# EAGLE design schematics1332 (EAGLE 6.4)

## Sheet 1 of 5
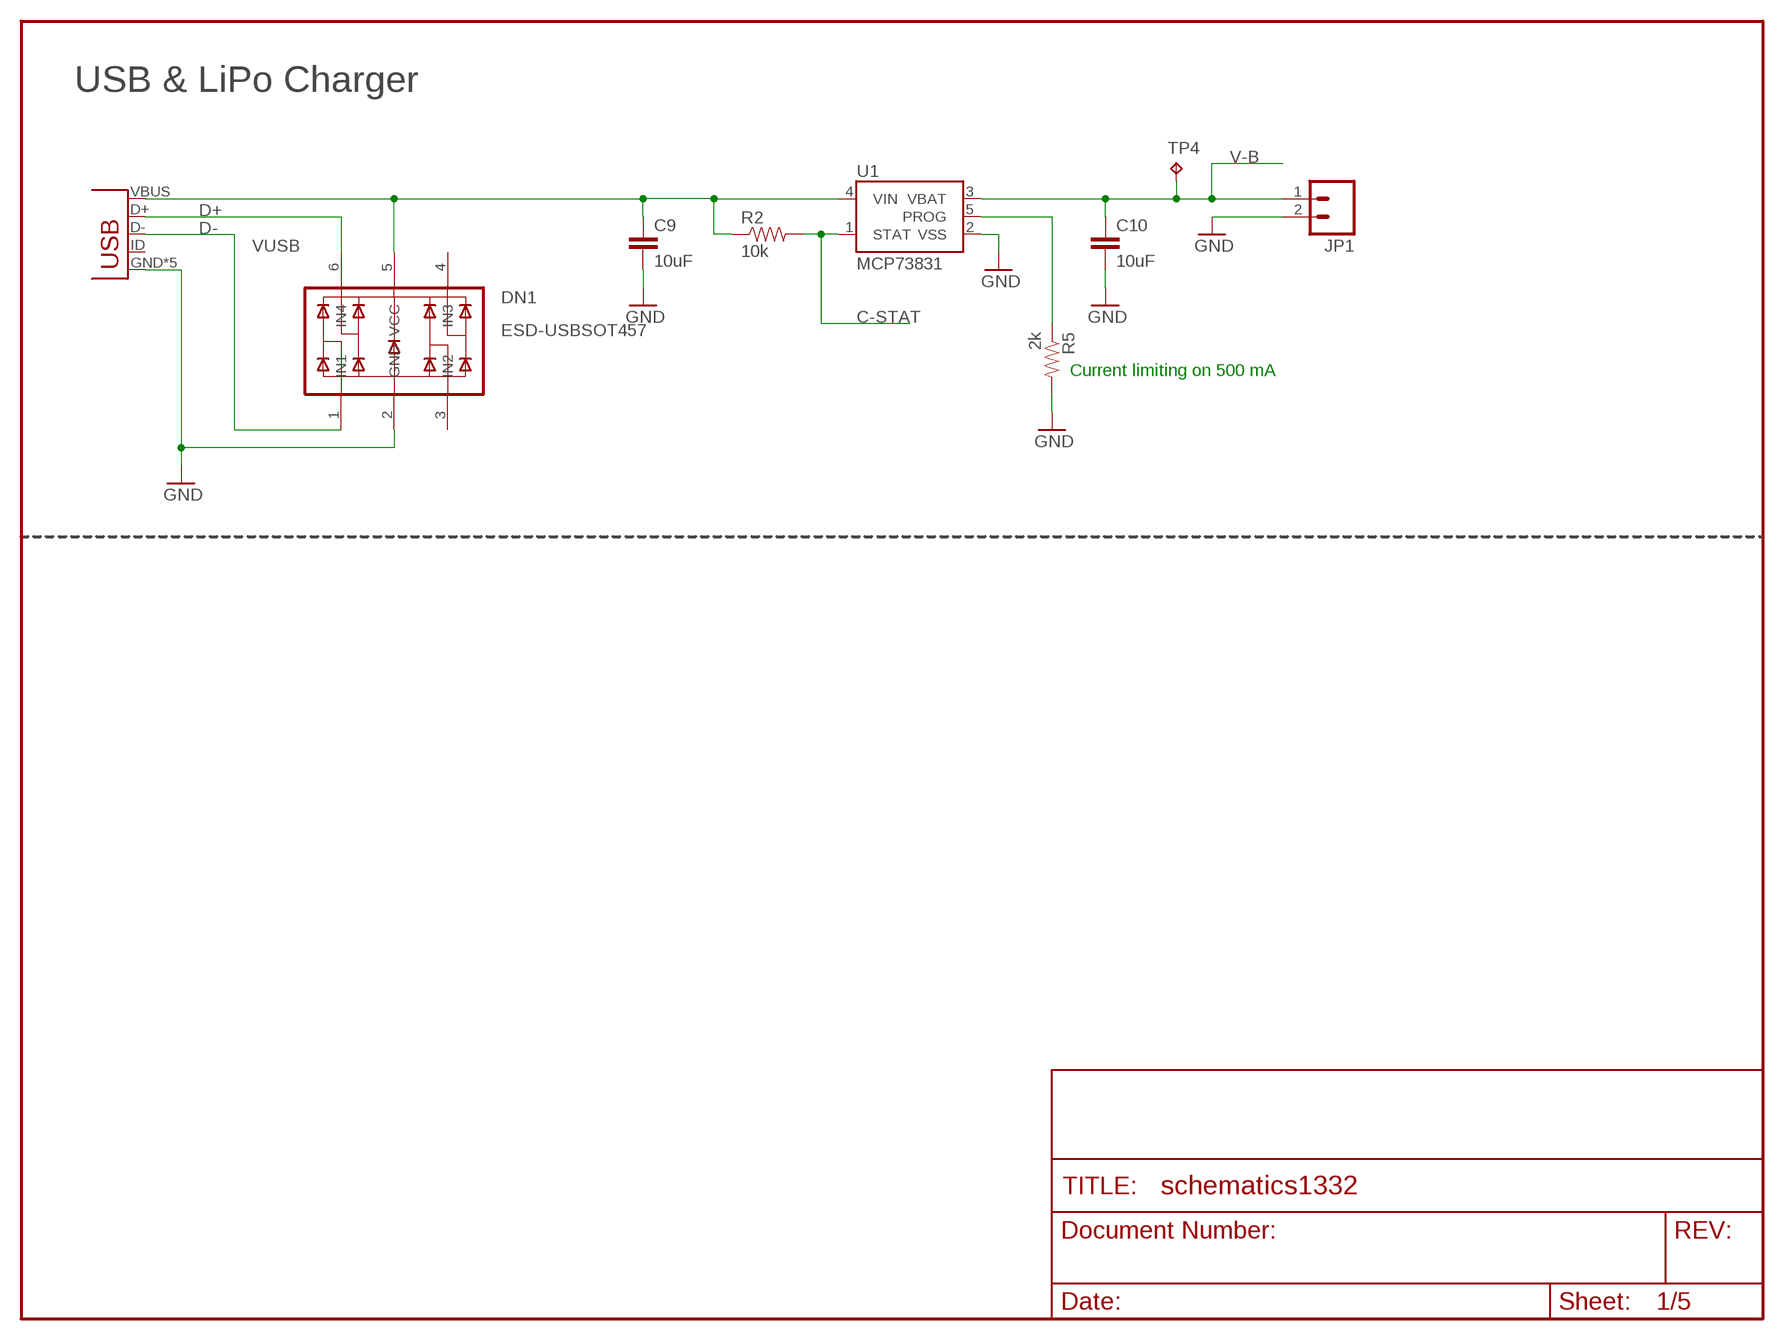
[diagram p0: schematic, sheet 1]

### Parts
C9  10uF  CAP0805  [0805]
C10  10uF  CAP0805  [0805]
DN1  ESD-USBSOT457  [SOT457]
JP1  M02-JST-2MM-SMT  [S2B-PH]
R2  10k  RESISTOR  [0805]
R5  2k  RESISTOR  [0805]
TP4  TPTP20R  [TP20R]
U1  MCP73831  [SOT23-5]
X1  USB  [MICRO-USB-B]

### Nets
C-STAT: R2.2 U1.1(STAT)
D+: DN1.6(IN4) X1.D+ ; also sheet 3
D-: DN1.1(IN1) X1.D- ; also sheet 3
GND: C9.2 C10.2 DN1.2(GND) JP1.2 R5.2 U1.2(VSS) X1.GND X1.GND@1(GND) X1.GND@2(GND) X1.GND@3(GND) X1.GND@4(GND) ; also sheet 2,3,4,5
N$11: R5.1 U1.5(PROG)
V-B: C10.1 JP1.1 TP4.TP U1.3(VBAT) ; also sheet 2
VUSB: C9.1 DN1.5(VCC) R2.1 U1.4(VIN) X1.VBUS ; also sheet 2
Unconnected: DN1.3(IN2) DN1.4(IN3) X1.ID

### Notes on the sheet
- USB & LiPo Charger
- Current limiting on 500 mA

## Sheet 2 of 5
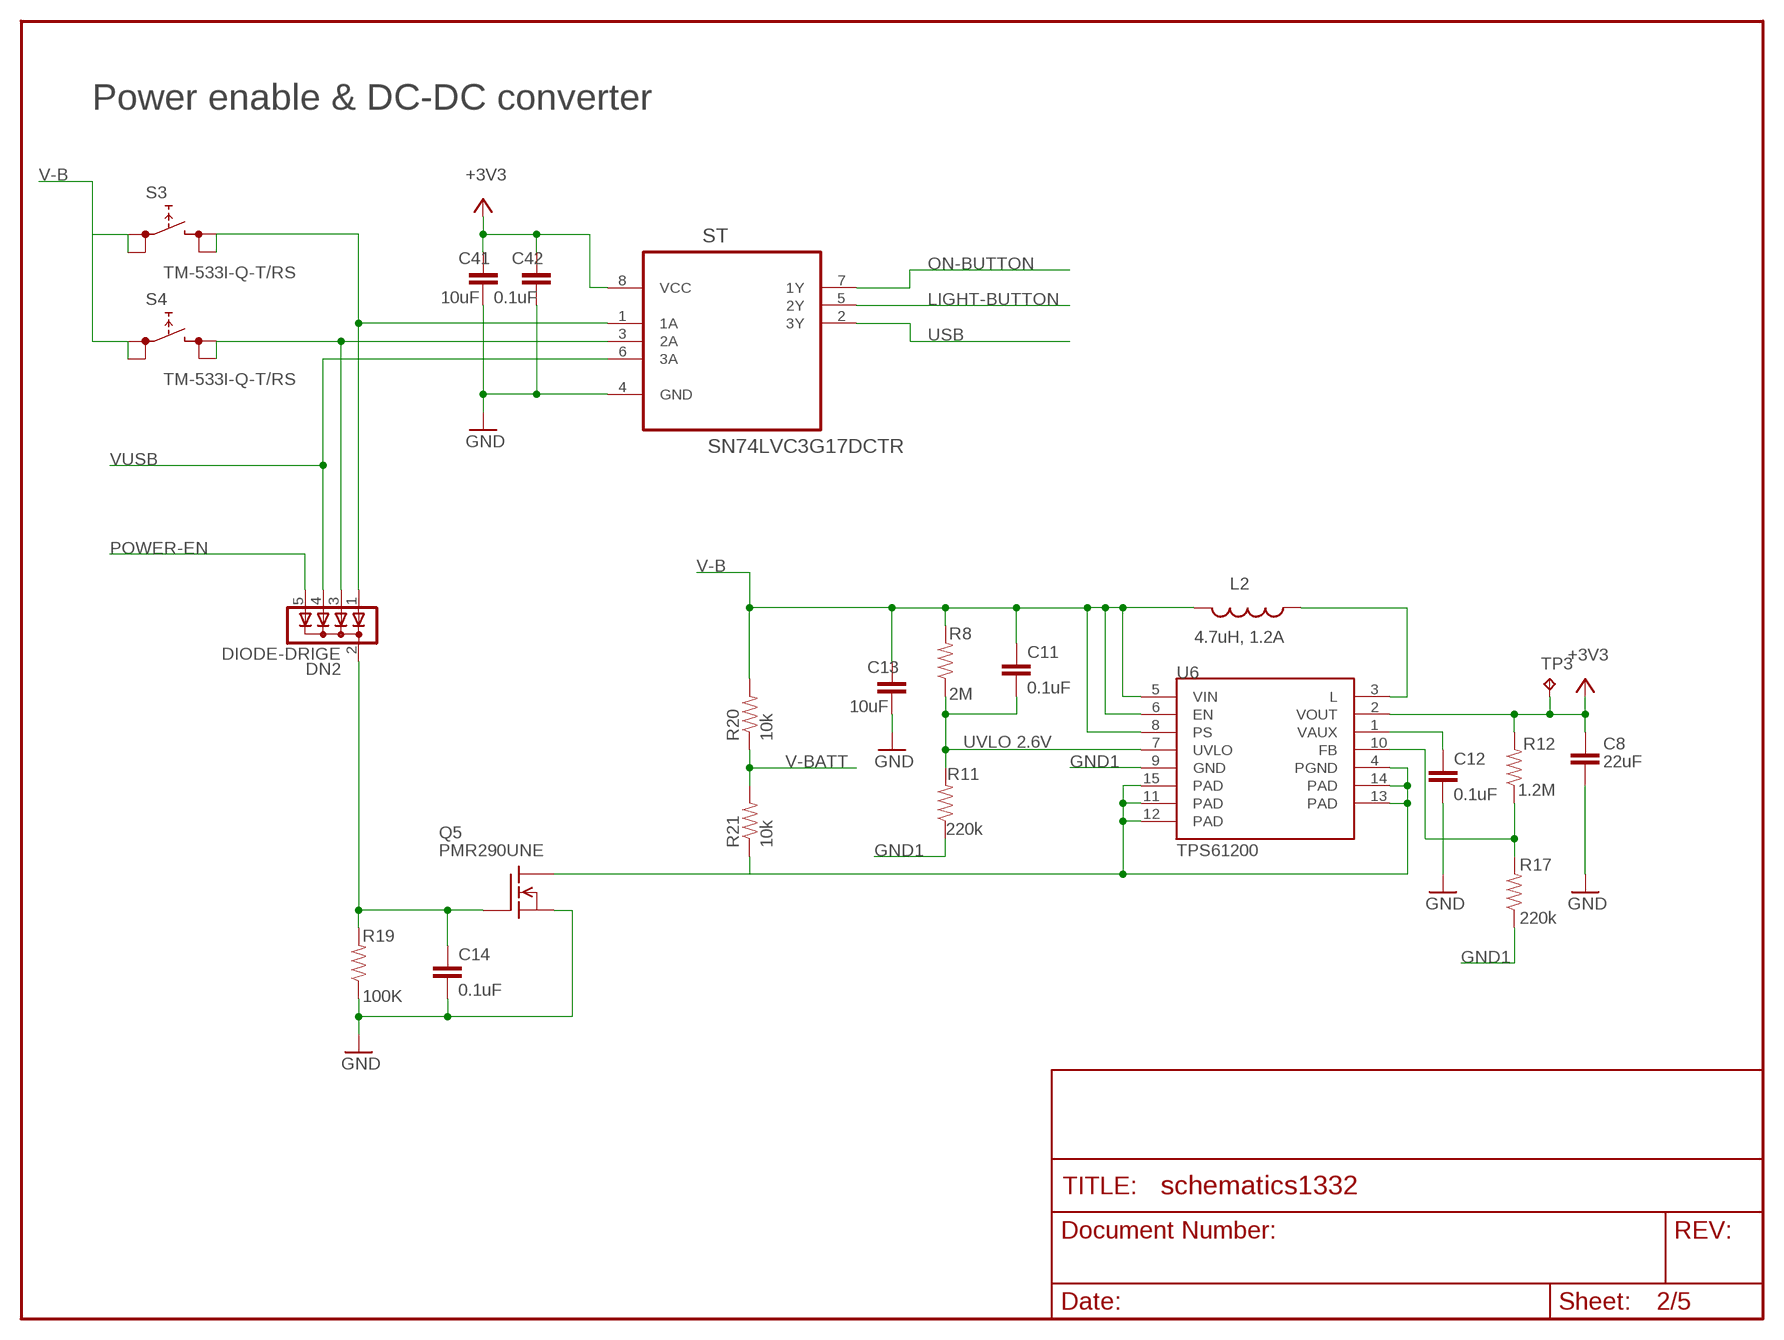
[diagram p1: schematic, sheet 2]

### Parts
C8  22uF  CAP0805  [0805]
C11  0.1uF  CAP0805  [0805]
C12  0.1uF  CAP0805  [0805]
C13  10uF  CAP0805  [0805]
C14  0.1uF  CAP0805  [0805]
C41  10uF  CAP0805  [0805]
C42  0.1uF  CAP0805  [0805]
DN2  DIODE-DRIGE  [SOT353]
L2  4.7uH, 1.2A  INDUCTOR.  [CDRH2D09]
Q5  PMR290UNE  [SOT23]
R8  2M  RESISTOR  [0805]
R11  220k  RESISTOR  [0805]
R12  1.2M  RESISTOR  [0805]
R17  220k  RESISTOR  [0805]
R19  100K  RESISTOR  [0805]
R20  10k  RESISTOR  [0805]
R21  10k  RESISTOR  [0805]
S3  TM-533I-Q-T/RS  [TM-533I-Q-T/R]
S4  TM-533I-Q-T/RS  [TM-533I-Q-T/R]
ST  SN74LVC3G17DCTR  [SOP65P400X130-8N]
TP3  TPTP20R  [TP20R]
U6  TPS61200  [QFN-10_PAD]

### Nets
3.3V1: R12.1 R17.2 U6.10(FB)
+3V3: C8.1 C41.1 C42.1 R12.2 ST.8(VCC) TP3.TP U6.2(VOUT) ; also sheet 3,4,5
GND: C8.2 C12.2 C13.2 C14.2 C41.2 C42.2 Q5.2(S) R19.1 ST.4(GND) ; also sheet 1,3,4,5
GND1: R11.1 R17.1 U6.9(GND)
LIGHT-BUTTON: ST.5(2Y)
LIGHT/WAKEUP-BUTTON1: DN2.3(A2) S4.T3 S4.T4 ST.3(2A)
N$8: L2.P$1 U6.3(L)
N$9: C12.1 U6.1(VAUX)
N$10: C14.1 DN2.2(C) Q5.1(G) R19.2
ON-BUTTON: ST.7(1Y)
PAD@4: Q5.3(D) R21.1 U6.4(PGND) U6.11(PAD) U6.12(PAD) U6.13(PAD) U6.14(PAD) U6.15(PAD)
POWER-EN: DN2.5(A4)
USB: ST.2(3Y)
UVLO1: C11.2 R8.1 R11.2 U6.7(UVLO)
V-B: C11.1 C13.1 L2.P$2 R8.2 R20.2 S3.T1 S3.T2 S4.T1 S4.T2 U6.5(VIN) U6.6(EN) U6.8(PS) ; also sheet 1
V-BATT: R20.1 R21.2 ; also sheet 3
VUSB: DN2.4(A3) ST.6(3A) ; also sheet 1
WAKEUP-BUTTON1: DN2.1(A1) S3.T3 S3.T4 ST.1(1A)

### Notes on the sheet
- Power enable & DC-DC converter
- UVLO 2.6V

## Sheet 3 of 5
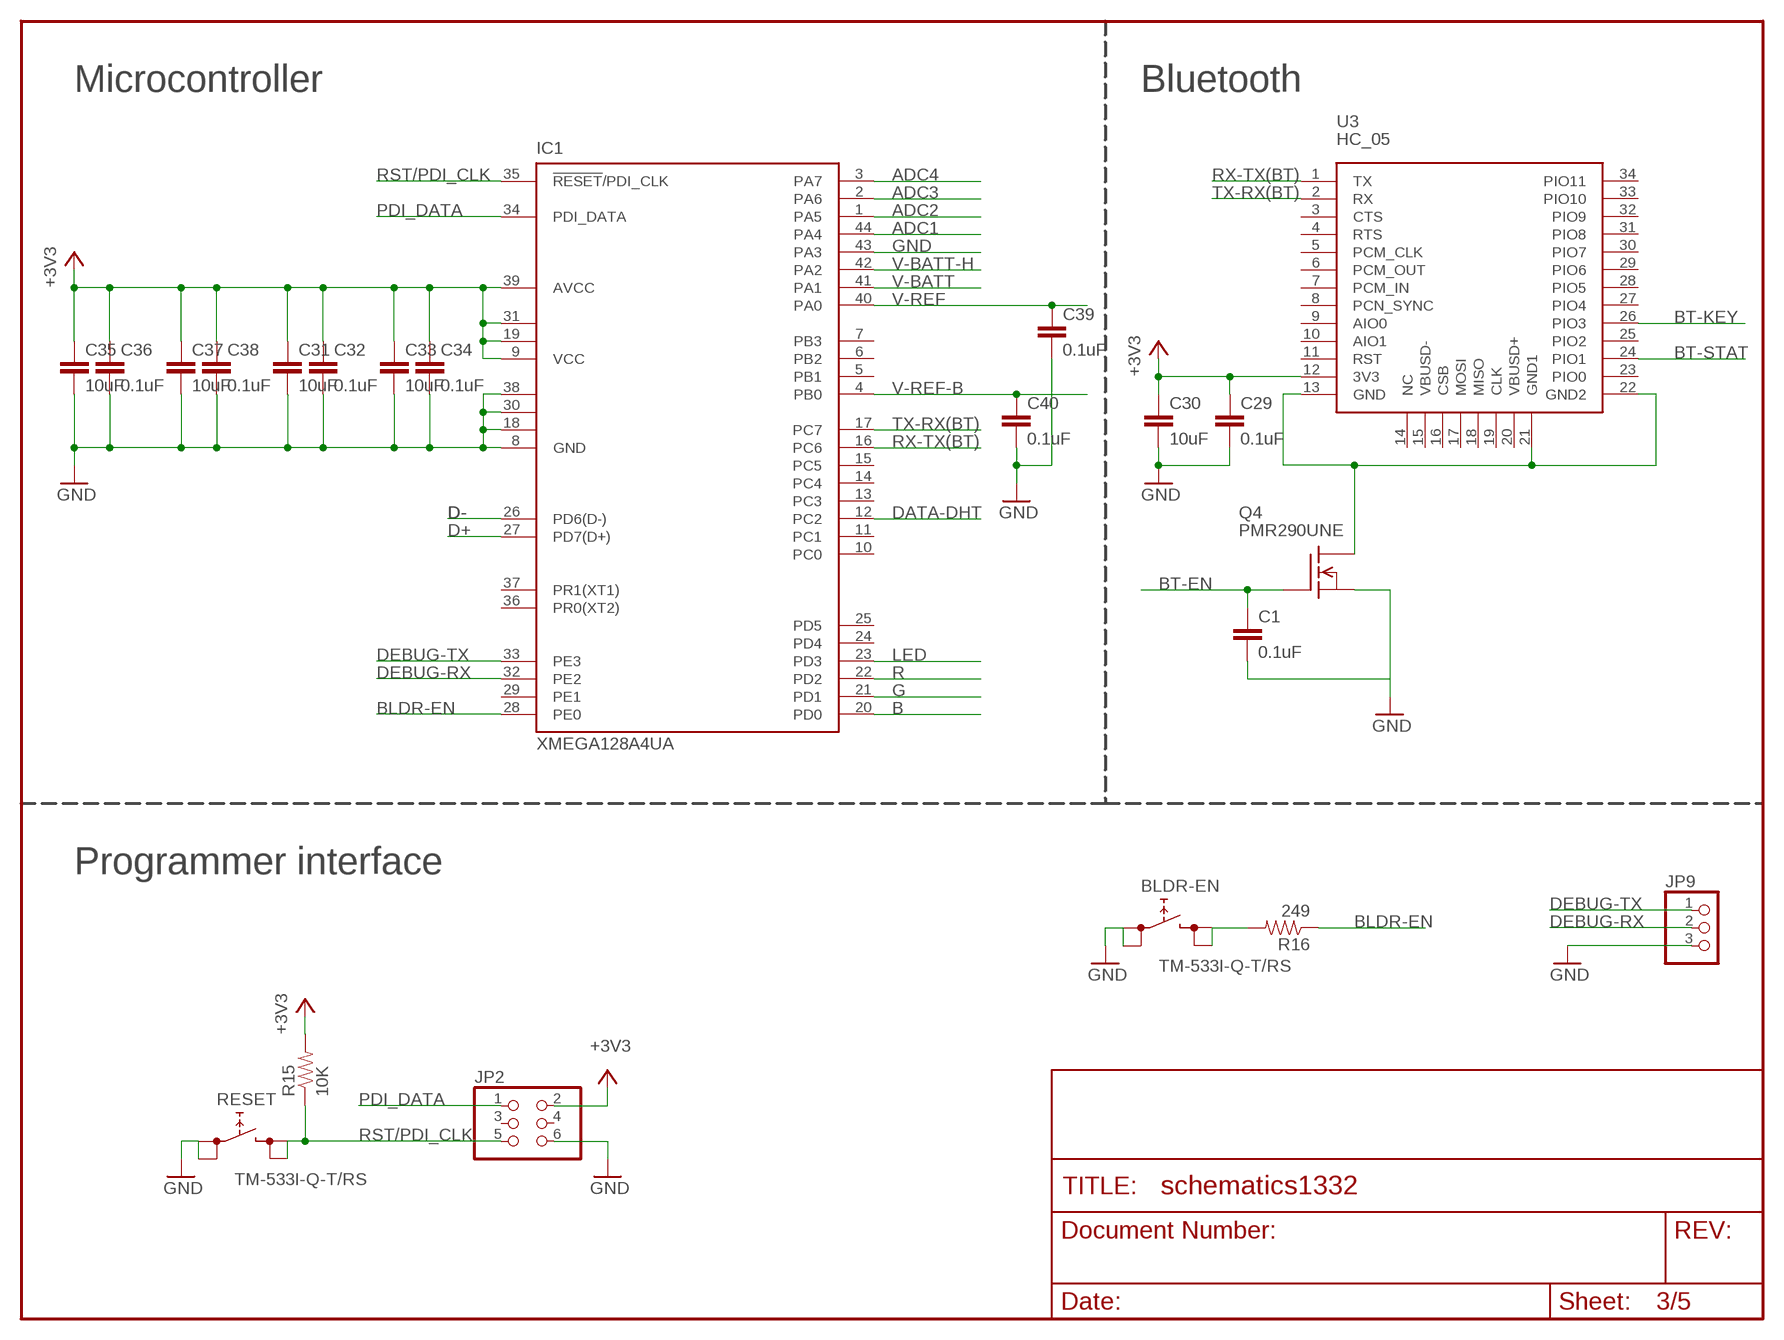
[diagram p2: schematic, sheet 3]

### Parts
BLDR-EN  TM-533I-Q-T/RS  [TM-533I-Q-T/R]
C1  0.1uF  CAP0805  [0805]
C29  0.1uF  CAP0805  [0805]
C30  10uF  CAP0805  [0805]
C31  10uF  CAP0805  [0805]
C32  0.1uF  CAP0805  [0805]
C33  10uF  CAP0805  [0805]
C34  0.1uF  CAP0805  [0805]
C35  10uF  CAP0805  [0805]
C36  0.1uF  CAP0805  [0805]
C37  10uF  CAP0805  [0805]
C38  0.1uF  CAP0805  [0805]
C39  0.1uF  CAP0805  [0805]
C40  0.1uF  CAP0805  [0805]
IC1  XMEGA128A4UA  [TQFP44]
JP2  PINHD-2X3  [2X03]
JP9  PINHD-1X3  [1X03]
Q4  PMR290UNE  [SOT23]
R15  10K  RESISTOR  [0805]
R16  249  RESISTOR  [0805]
RESET  TM-533I-Q-T/RS  [TM-533I-Q-T/R]
U3  HC_05  [BLUETOOTH_SMD]

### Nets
+3V3: C29.1 C30.1 C31.1 C32.1 C33.1 C34.1 C35.1 C36.1 C37.1 C38.1 IC1.9(VCC) IC1.19(VCC1) IC1.31(VCC2) IC1.39(AVCC) JP2.2 R15.2 U3.12(3V3) ; also sheet 2,4,5
ADC1: IC1.44(PA4) ; also sheet 4
ADC2: IC1.1(PA5) ; also sheet 4
ADC3: IC1.2(PA6) ; also sheet 4
ADC4: IC1.3(PA7) ; also sheet 4
B: IC1.20(PD0) ; also sheet 5
BLDR-EN: IC1.28(PE0) R16.1
BT-EN: C1.1 Q4.1(G)
BT-KEY: U3.26(PIO3)
BT-STAT: U3.24(PIO1)
D+: IC1.27(PD7(D+)) ; also sheet 1
D-: IC1.26(PD6(D-)) ; also sheet 1
DATA-DHT: IC1.12(PC2) ; also sheet 5
DEBUG-RX: IC1.32(PE2) JP9.2
DEBUG-TX: IC1.33(PE3) JP9.1
G: IC1.21(PD1) ; also sheet 5
GND: BLDR-EN.T1 BLDR-EN.T2 C1.2 C29.2 C30.2 C31.2 C32.2 C33.2 C34.2 C35.2 C36.2 C37.2 C38.2 C39.2 C40.2 IC1.8(GND) IC1.18(GND1) IC1.30(GND2) IC1.38(GND3) IC1.43(PA3) JP2.6 JP9.3 Q4.2(S) RESET.T1 RESET.T2 ; also sheet 1,2,4,5
LED: IC1.23(PD3) ; also sheet 5
N$4: Q4.3(D) U3.13(GND) U3.21(GND1) U3.22(GND2)
N$5: BLDR-EN.T3 BLDR-EN.T4 R16.2
PDI_DATA: IC1.34(PDI_DATA) JP2.1
R: IC1.22(PD2) ; also sheet 5
RST/PDI_CLK: IC1.35(!RESET!/PDI_CLK) JP2.5 R15.1 RESET.T3 RESET.T4
RX-TX(BT): IC1.16(PC6) U3.1(TX)
TX-RX(BT): IC1.17(PC7) U3.2(RX)
V-BATT: IC1.41(PA1) ; also sheet 2
V-BATT-H: IC1.42(PA2) ; also sheet 4
V-REF: C39.1 IC1.40(PA0) ; also sheet 4
V-REF-B: C40.1 IC1.4(PB0) ; also sheet 4
Unconnected: IC1.5(PB1) IC1.6(PB2) IC1.7(PB3) IC1.10(PC0) IC1.11(PC1) IC1.13(PC3) IC1.14(PC4) IC1.15(PC5) IC1.24(PD4) IC1.25(PD5) IC1.29(PE1) IC1.36(PR0(XT2)) IC1.37(PR1(XT1)) JP2.3 JP2.4 U3.3(CTS) U3.4(RTS) U3.5(PCM_CLK) U3.6(PCM_OUT) U3.7(PCM_IN) U3.8(PCN_SYNC) U3.9(AIO0) U3.10(AIO1) U3.11(RST) U3.14(NC) U3.15(VBUSD-) U3.16(CSB) U3.17(MOSI) U3.18(MISO) U3.19(CLK) U3.20(VBUSD+) U3.23(PIO0) U3.25(PIO2) U3.27(PIO4) U3.28(PIO5) U3.29(PIO6) U3.30(PIO7) U3.31(PIO8) U3.32(PIO9) U3.33(PIO10) U3.34(PIO11)

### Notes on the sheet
- Microcontroller | Bluetooth
- Programmer interface

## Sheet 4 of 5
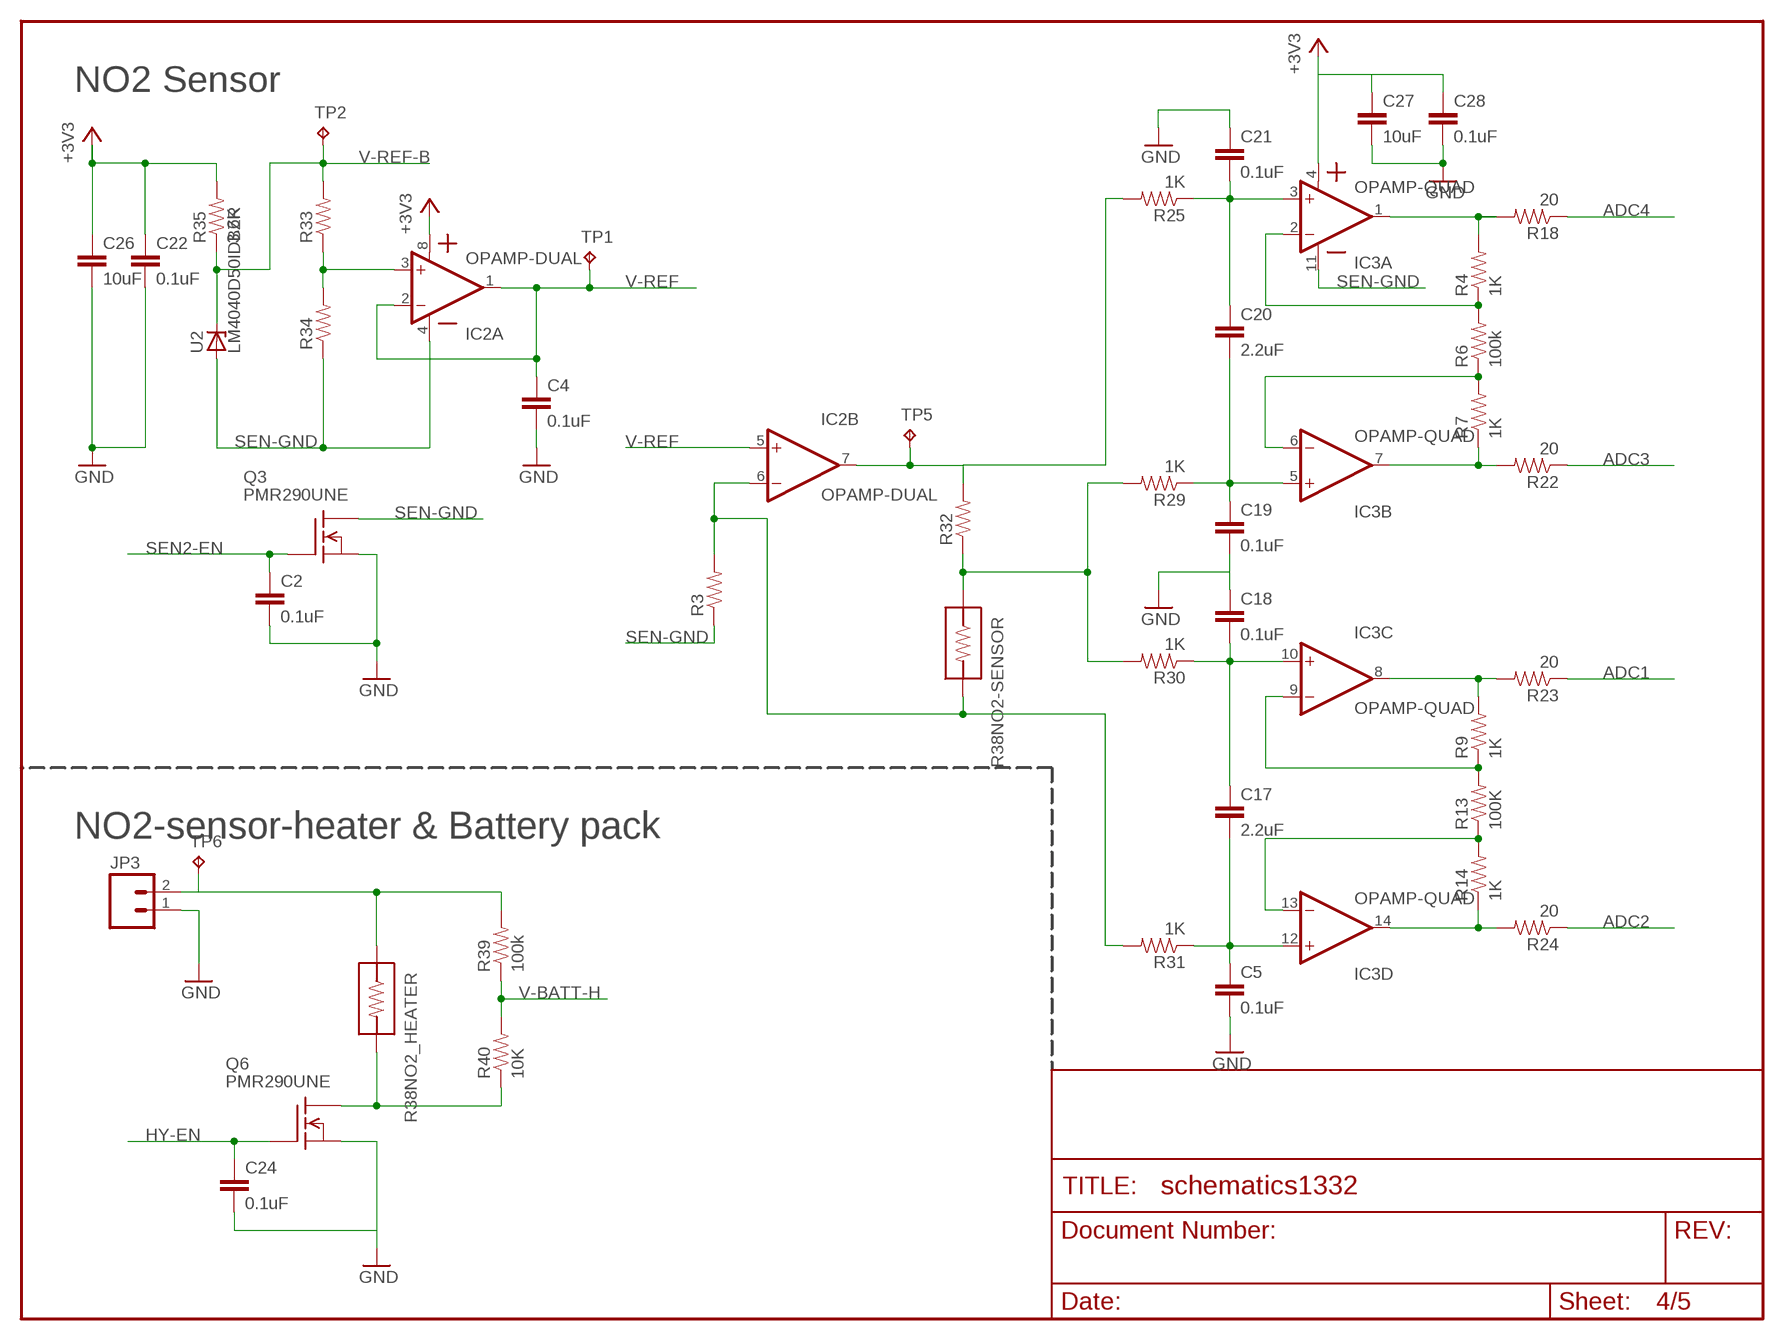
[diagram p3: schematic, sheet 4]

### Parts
C2  0.1uF  CAP0805  [0805]
C4  0.1uF  CAP0805  [0805]
C5  0.1uF  CAP0805  [0805]
C17  2.2uF  CAP0805  [0805]
C18  0.1uF  CAP0805  [0805]
C19  0.1uF  CAP0805  [0805]
C20  2.2uF  CAP0805  [0805]
C21  0.1uF  CAP0805  [0805]
C22  0.1uF  CAP0805  [0805]
C24  0.1uF  CAP0805  [0805]
C26  10uF  CAP0805  [0805]
C27  10uF  CAP0805  [0805]
C28  0.1uF  CAP0805  [0805]
IC2  OPAMP-DUAL  [SOIC127P600X175-8N]
IC3  OPAMP-QUAD  [SOIC127P600X175-14N]
JP3  M025MM  [SCREWTERMINAL-5MM-2]
Q3  PMR290UNE  [SOT23]
Q6  PMR290UNE  [SOT23]
R3  RESISTOR  [0805]
R4  1K  RESISTOR  [0805]
R6  100k  RESISTOR  [0805]
R7  1K  RESISTOR  [0805]
R9  1K  RESISTOR  [0805]
R13  100K  RESISTOR  [0805]
R14  1K  RESISTOR  [0805]
R18  20  RESISTOR  [0805]
R22  20  RESISTOR  [0805]
R23  20  RESISTOR  [0805]
R24  20  RESISTOR  [0805]
R25  1K  RESISTOR  [0805]
R29  1K  RESISTOR  [0805]
R30  1K  RESISTOR  [0805]
R31  1K  RESISTOR  [0805]
R32  RESISTOR  [0805]
R33  RESISTOR  [0805]
R34  RESISTOR  [0805]
R35  3.6K  RESISTOR  [0805]
R38  NO2-SENSOR  [DIP08]
R39  100k  RESISTOR  [0805]
R40  10K  RESISTOR  [0805]
TP1  TPTP20R  [TP20R]
TP2  TPTP20R  [TP20R]
TP5  TPTP20R  [TP20R]
TP6  TPTP20R  [TP20R]
U2  LM4040D50IDBZR  [SOT95P237X112-3N]

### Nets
+3V3: C22.1 C26.1 C27.1 C28.1 IC2.8(A:VDD) IC3.4(A:VDD) R35.2 ; also sheet 2,3,5
ADC1: R23.1 ; also sheet 3
ADC2: R24.1 ; also sheet 3
ADC3: R22.1 ; also sheet 3
ADC4: R18.1 ; also sheet 3
GND: C2.2 C4.2 C5.2 C18.1 C19.2 C21.1 C22.2 C24.2 C26.2 C27.2 C28.2 JP3.1 Q3.2(S) Q6.2(S) ; also sheet 1,2,3,5
HY-EN: C24.1 Q6.1(G)
N$1: IC3.2(A:-IN) R4.1 R6.2
N$2: IC3.6(B:-IN) R6.1 R7.2
N$7: IC3.9(C:-IN) R9.1 R13.2
N$12: IC3.13(D:-IN) R13.1 R14.2
N$14: IC3.1(A:OUT) R4.2 R18.2
N$15: IC3.7(B:OUT) R7.1 R22.2
N$19: IC3.8(C:OUT) R9.2 R23.2
N$21: IC3.14(D:OUT) R14.1 R24.2
N$22: C17.1 C18.2 IC3.10(C:+IN) R30.1
N$23: IC2.3(A:+IN) R33.1 R34.2
N$25: C19.1 C20.2 IC3.5(B:+IN) R29.1
N$26: C20.1 C21.2 IC3.3(A:+IN) R25.1
N$27: C5.1 C17.2 IC3.12(D:+IN) R31.1
N$28: JP3.2 R38.2 R39.2 TP6.TP
N$29: Q6.3(D) R38.7 R40.1
N$33: R29.2 R30.2 R32.1 R38.1
N$34: IC2.7(B:OUT) R25.2 R32.2 TP5.TP
N$35: IC2.6(B:-IN) R3.2 R31.2 R38.8
SEN2-EN: C2.1 Q3.1(G)
SEN-GND: IC2.4(A:GND) IC3.11(A:GND) Q3.3(D) R3.1 R34.1 U2.2(A)
V-BATT-H: R39.1 R40.2 ; also sheet 3
V-REF: C4.1 IC2.1(A:OUT) IC2.2(A:-IN) IC2.5(B:+IN) TP1.TP ; also sheet 3
V-REF-B: R33.2 R35.1 TP2.TP U2.1(C) ; also sheet 3

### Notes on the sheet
- NO2 Sensor
- NO2-sensor-heater & Battery pack

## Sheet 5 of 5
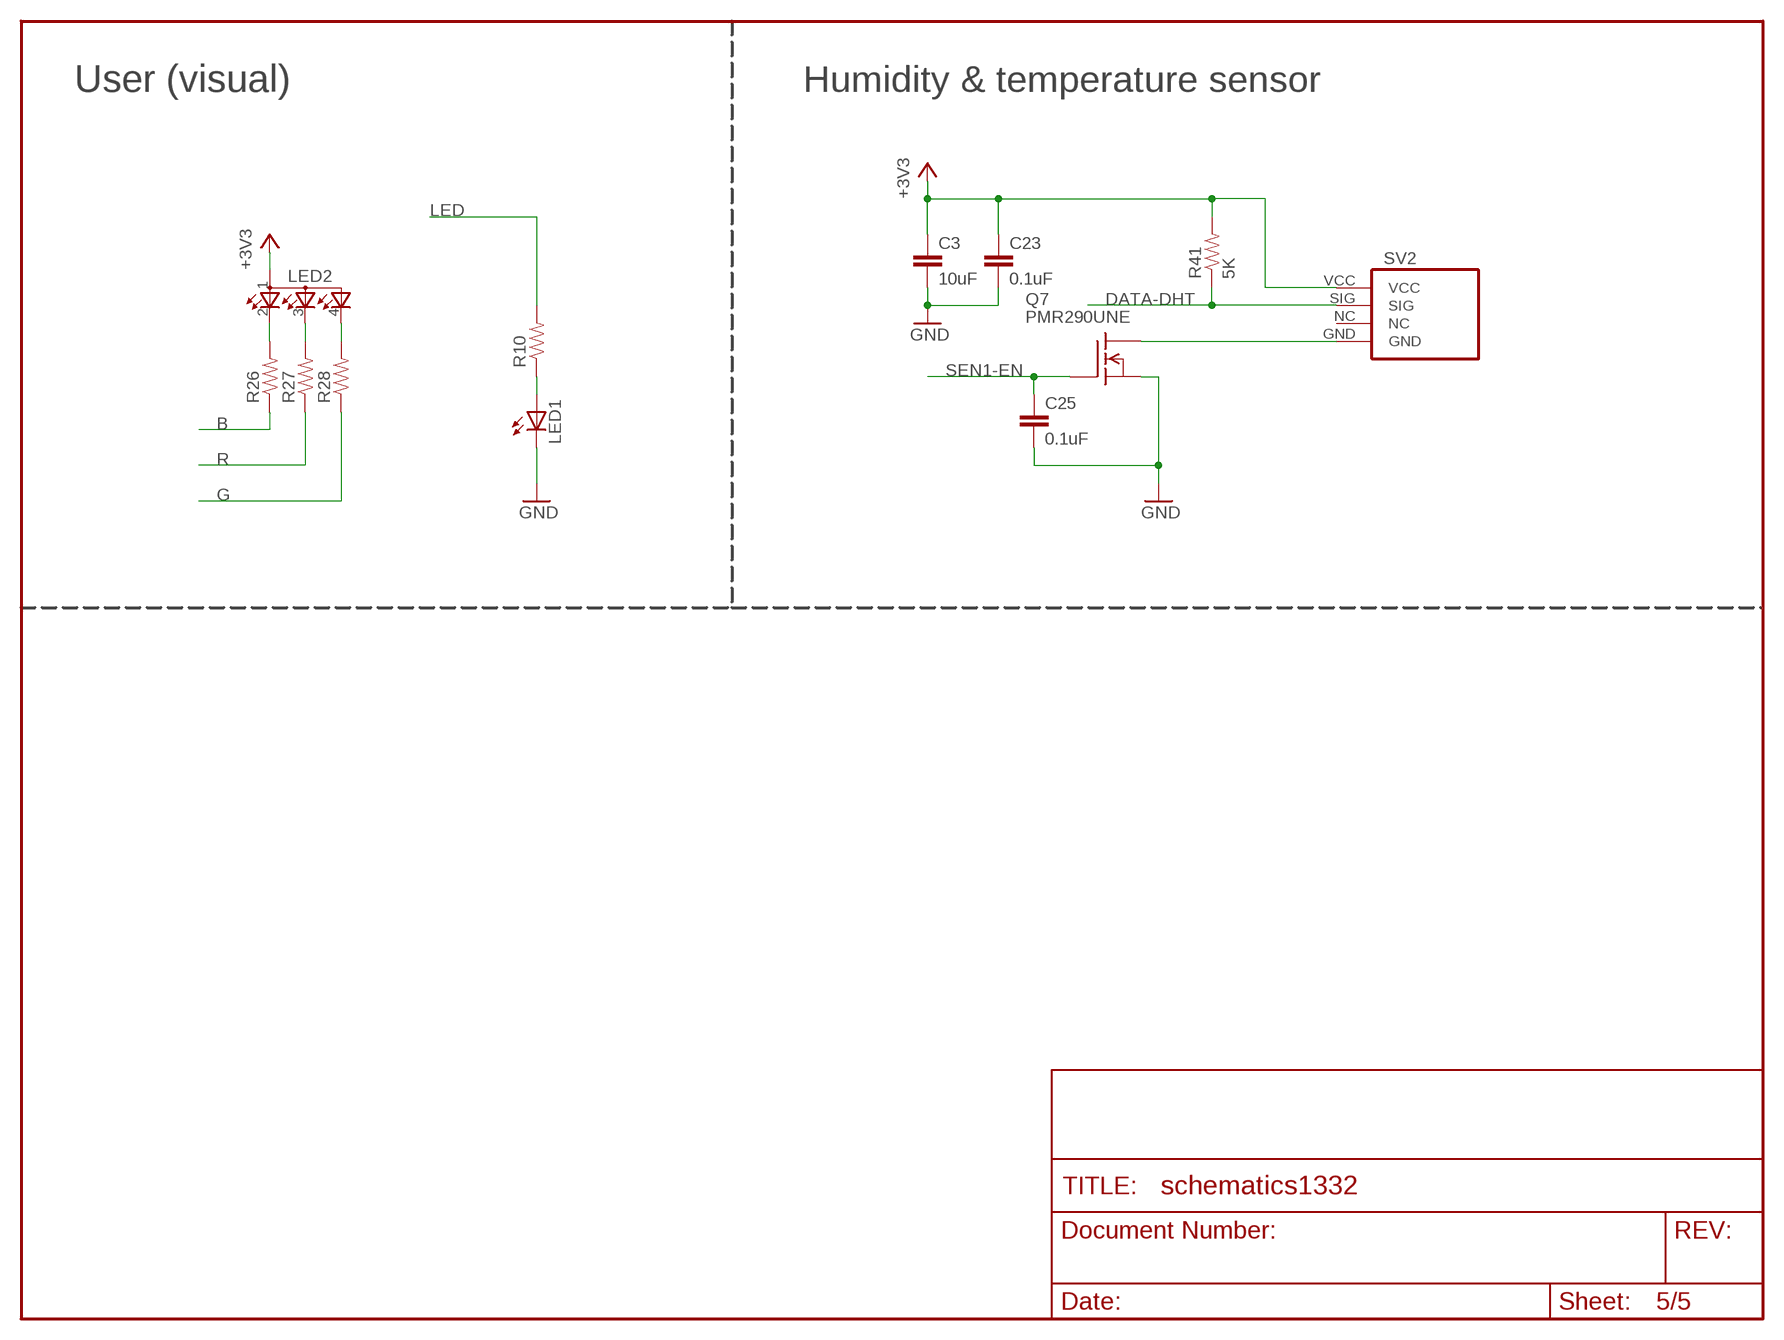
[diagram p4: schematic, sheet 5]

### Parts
C3  10uF  CAP0805  [0805]
C23  0.1uF  CAP0805  [0805]
C25  0.1uF  CAP0805  [0805]
LED1  LED5MM  [LED5MM]
LED2  RGBLED  [150141M173100]
Q7  PMR290UNE  [SOT23]
R10  RESISTOR  [0805]
R26  RESISTOR  [0805]
R27  RESISTOR  [0805]
R28  RESISTOR  [0805]
R41  5K  RESISTOR  [0805]
SV2  DHT11  [DHT11]

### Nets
435: LED2.3(3R) R27.2
+3V3: C3.1 C23.1 LED2.1 R41.2 SV2.VCC ; also sheet 2,3,4
B: R26.1 ; also sheet 3
B2: LED2.2(2B) R26.2
DATA-DHT: R41.1 SV2.SIG ; also sheet 3
G: R28.1 ; also sheet 3
G2: LED2.4(4G) R28.2
GND: C3.2 C23.2 C25.2 LED1.K(C) Q7.2(S) ; also sheet 1,2,3,4
LED: R10.2 ; also sheet 3
N$6: LED1.A R10.1
N$30: Q7.3(D) SV2.GND
R: R27.1 ; also sheet 3
SEN1-EN: C25.1 Q7.1(G)
Unconnected: SV2.NC

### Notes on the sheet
- User (visual) | Humidity & temperature sensor

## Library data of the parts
BLDR-EN RESET S3 S4 = snuffelneus:TM-533I-Q-T/R: 6.2 X 6.5mm TACT Switch (SMD) Source: http://www3.alps.co.jp/WebObjects/catalog.woa/PDF/E/Switch/Tact/SKHM/SKHM.PDF
C1-C5 C9-C12 C14 C17-C40 = SparkFun:CAP: Capacitor
C8 C13 C41 C42 = CH_passive:CAP: Capacitor
DN1 = snuffelneus:ESD-USB: 4 DIODES SIL, common cathode
DN2 = snuffelneus:DIODE-DRIGE: 4 DIODES SIL, common cathode
IC1 = snuffelneus:XMEGA128A4U: MICROCONTROLLER Features High-performance, Low-power 8/16-bit AVR XMEGA Microcontroller Non-Volatile Program and Data Memories - 16 KB - 128 KB of In-System Self-Programmable Flash - 4 KB - 8 KB Boot Code Section with Independent Lock Bits - 1 KB - 2 KB EEPROM - 2 KB - 8 KB Internal SRAM Peripheral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; OC_FARNELL: unknown; OC_NEWARK: unknown
IC2 = snuffelneus:OPAMP-DUAL: Operational Amplifier
IC3 = snuffelneus:OPAMP-QUAD: Operational Amplifier
JP1 JP3 = SparkFun:M02: Header 2
JP2 = pinhead:PINHD-2X3: PIN HEADER
JP9 = pinhead:PINHD-1X3: PIN HEADER
L2 = SparkFun:INDUCTOR: Inductors
LED1 = led:LED: LED
LED2 = snuffelneus:RGBLED: OSRAM - Hyper Multi TOPLED® (RGB) LB E673, LV E673, LT E673 - Power TOPLED® Enhanced optical Power LED (HOP2000) LS E67B, LA E67B, LO E67B, LY E67B - Hyper Multi TOPLED® Enhanced optical Power LED (HOP2000 / ATON®) LATB T66B - Hyper Multi TOPLED® Hyper-Bright LED LATB T686 Source: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
Q3-Q7 = snuffelneus:PMR290UNE: N-Channel Enhancement MOSFET 200V; 1.5A; 1,6Ohm
R2-R35 R39-R41 = SparkFun:RESISTOR: Resistor
R38 = snuffelneus:NO2-SENSOR: Resistor Basic schematic elements and footprints for 0603, 1206, and PTH 1/10th watt (small) resistors.
ST = snuffelneus:SN74LVC3G17DCTR: TRIPLE SCHMITT-TRIGGER BUFFER; MPN: SN74LVC3G17DCTR; OC_FARNELL: 1236391; OC_NEWARK: 90H3713; PACKAGE: SSOP-8; SUPPLIER: Texas Instruments
SV2 = snuffelneus:DHT11: PIN HEADER
TP1-TP6 = testpad:TP: Test pad
U1 = SparkFun:MCP73831: Microchip's MCP73831 Miniature single cell, fully integrated Li-Ion, Li-polymer charge management controller http://ww1.microchip.com/downloads/en/DeviceDoc/21984a.pdf
U2 = snuffelneus:LM4040D50IDBZR: PRECISION MICROPOWER SHUNT VOLTAGE REFERENCE; MPN: LM4040D50IDBZR; OC_FARNELL: 1652239; OC_NEWARK: 43K3367; PACKAGE: 3-SOT-23; SUPPLIER: TEXAS INSTRUMENTS
U3 = SerialPortBluetooth:HC_05
U6 = SparkFun:TPS61200: DC to DC Booster
X1 = snuffelneus:USB: USB Connectors USB-B-PTH is fully proven SKU : PRT-00139 USB-miniB is fully proven SKU : PRT-00587 USB-A-PCB is untested. USB-A-H is throughly reviewed, but untested. Spark Fun Electronics SKU : PRT-00437 USB-B-SMT is throughly reviewed, but untested. Needs silkscreen touching up. USB-A-S has not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

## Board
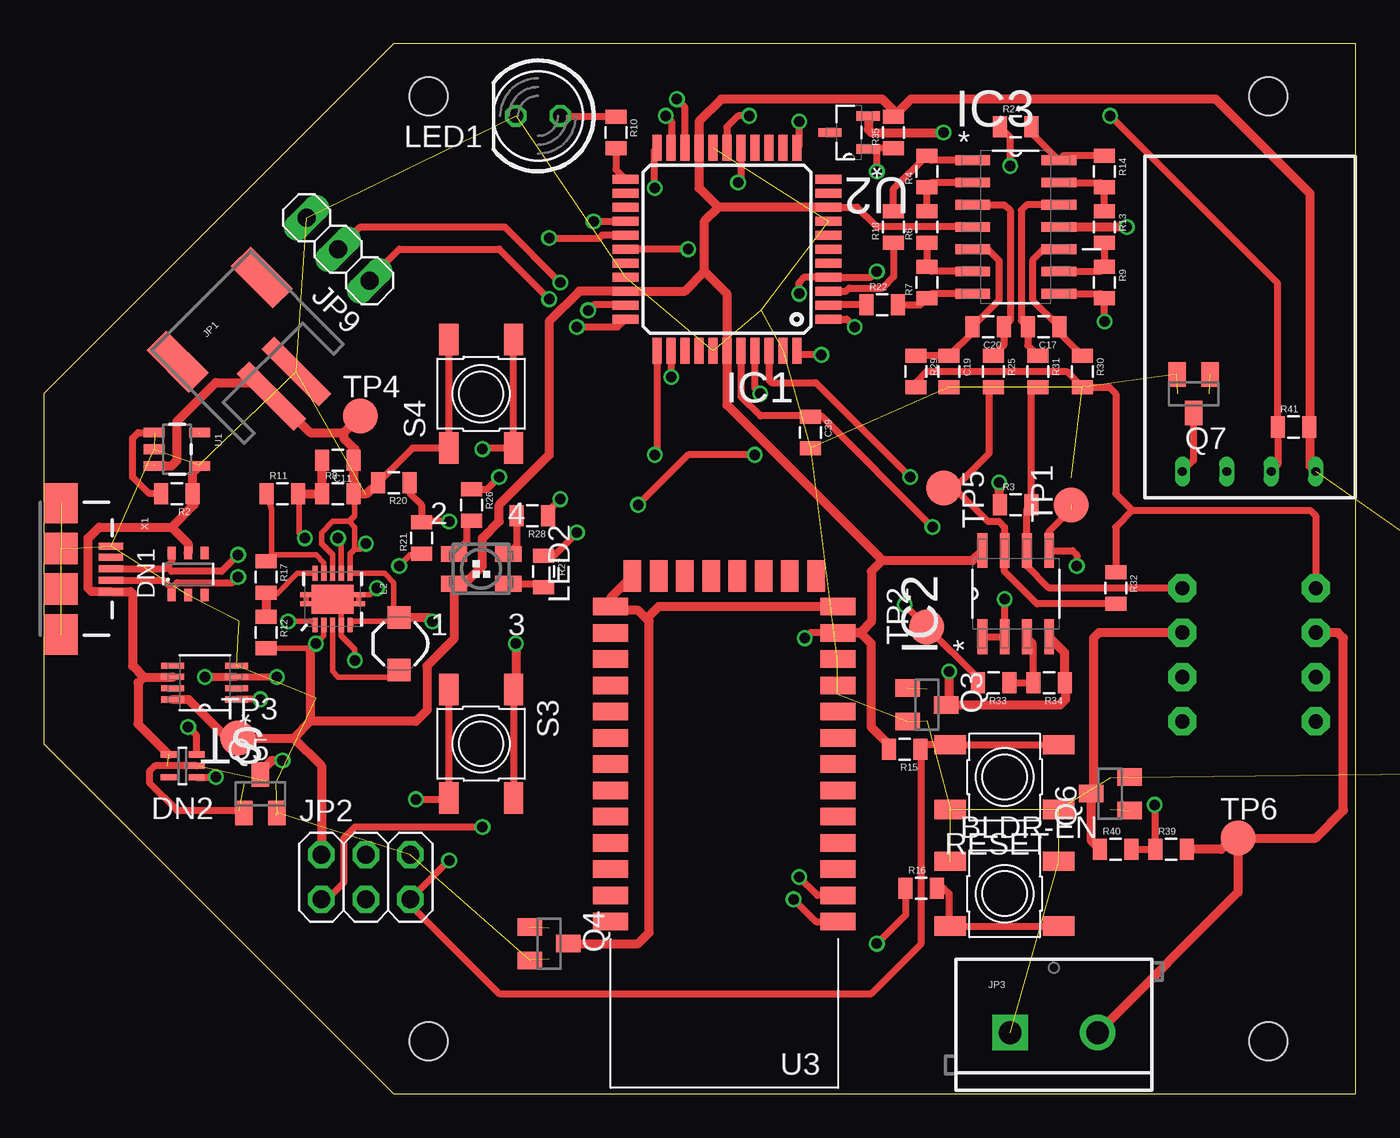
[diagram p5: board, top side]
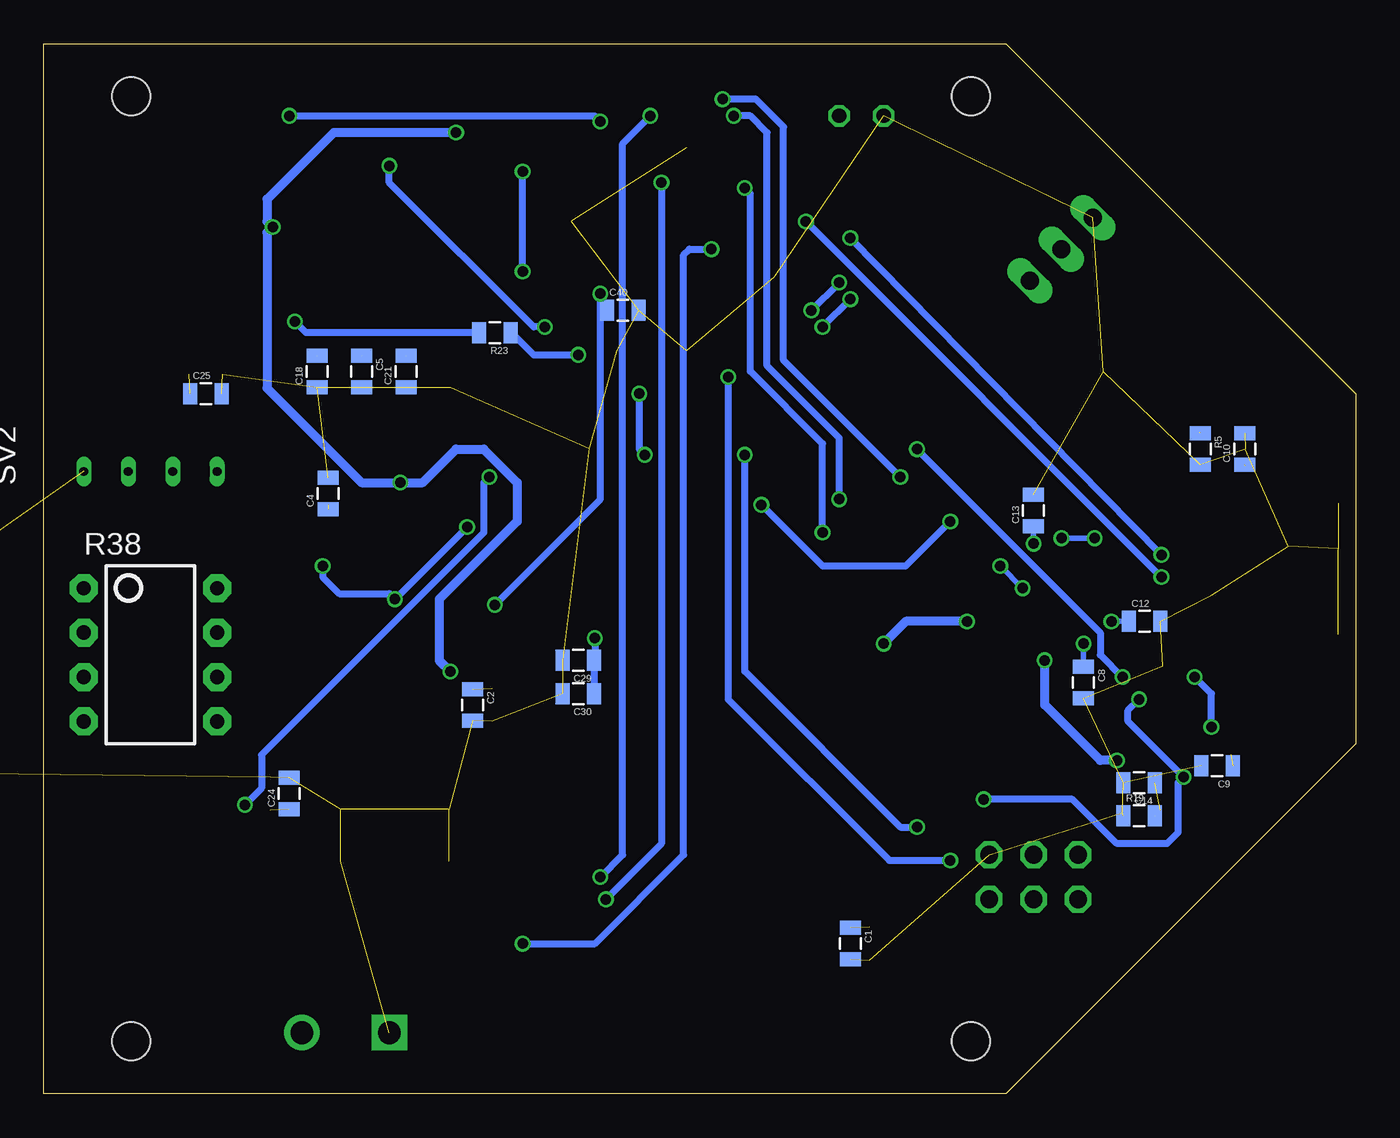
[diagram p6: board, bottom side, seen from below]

Size 75 x 60 mm. Coordinates in mm from the lower left corner, seen from the top.
Outline: 0,20 20,0 75,0 75,60 20,60 0,40 0,20
Copper layers (1*16): Top 0.018mm / dielectric 1.55mm / Bottom 0.018mm
Design rules "eC_2Layer_PClass6_BaseCopperO18_eCDefault": minimum track width 0.15mm, minimum drill 0.35mm, track to track 0.15mm, track to pad 0.15mm, pad to pad 0.15mm, via to via 0.15mm, smd to smd 0mil, copper to edge 0.25mm, drill to drill 0.35mm, minimum pad ring 0.175mm, minimum via ring 0.125mm, stop-mask expansion 0mil, vias tented up to drill 0.45mm, thermal gap 0.2mm
Holes 2.2 mm at 70,57 22,57 22,3 70,3
tRestrict: area 62.9,18.1 to 74.9,32.7
bRestrict: area 62.9,18.1 to 74.9,32.7

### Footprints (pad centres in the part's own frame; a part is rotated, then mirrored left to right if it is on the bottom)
TM-533I-Q-T/R = smd 1.8 x 1.1: T1 -3.1,1.85; T2 3.1,1.85; T3 -3.1,-1.85; T4 3.1,-1.85
0805 = smd 0.8 x 1.2: 1 -0.9,0; 2 0.9,0
SOT457 = smd 0.7 x 0.45: 1 -1.2,0.95; 2 -1.2,0; 3 -1.2,-0.95; 4 1.2,-0.95; 5 1.2,0; 6 1.2,0.95
SOT353 = smd 0.35 x 0.9: 1 -0.65,-0.8; 2 0,-0.8; 3 0.65,-0.8; 4 0.65,0.8; 5 -0.65,0.8
TQFP44 = smd 1.5 x 0.5: 1 -5.8,4; 2 -5.8,3.2; 3 -5.8,2.4; 4 -5.8,1.6; 5 -5.8,0.8; 6 -5.8,0; 7 -5.8,-0.8; 8 -5.8,-1.6; 9 -5.8,-2.4; 10 -5.8,-3.2; 11 -5.8,-4; 23 5.8,-4; 24 5.8,-3.2; 25 5.8,-2.4; 26 5.8,-1.6; 27 5.8,-0.8; 28 5.8,0; 29 5.8,0.8; 30 5.8,1.6; 31 5.8,2.4; 32 5.8,3.2; 33 5.8,4 | smd 0.5 x 1.5: 12 -4,-5.8; 13 -3.2,-5.8; 14 -2.4,-5.8; 15 -1.6,-5.8; 16 -0.8,-5.8; 17 0,-5.8; 18 0.8,-5.8; 19 1.6,-5.8; 20 2.4,-5.8; 21 3.2,-5.8; 22 4,-5.8; 34 4,5.8; 35 3.2,5.8; 36 2.4,5.8; 37 1.6,5.8; 38 0.8,5.8; 39 0,5.8; 40 -0.8,5.8; 41 -1.6,5.8; 42 -2.4,5.8; 43 -3.2,5.8; 44 -4,5.8
SOIC127P600X175-8N = smd 1.981 x 0.559: 1 -2.464,1.905; 2 -2.464,0.635; 3 -2.464,-0.635; 4 -2.464,-1.905; 5 2.464,-1.905; 6 2.464,-0.635; 7 2.464,0.635; 8 2.464,1.905
SOIC127P600X175-14N = smd 1.981 x 0.559: 1 -2.464,3.81; 2 -2.464,2.54; 3 -2.464,1.27; 4 -2.464,0; 5 -2.464,-1.27; 6 -2.464,-2.54; 7 -2.464,-3.81; 8 2.464,-3.81; 9 2.464,-2.54; 10 2.464,-1.27; 11 2.464,0; 12 2.464,1.27; 13 2.464,2.54; 14 2.464,3.81
S2B-PH = smd 1 x 4.6: 1 -1,-3.7; 2 1,-3.7 | smd 1.6 x 3.4: NC1 -3.4,1.5; NC2 3.4,1.5
2X03 = drill 1.016 octagon: 1 -2.54,-1.27; 2 -2.54,1.27; 3 0,-1.27; 4 0,1.27; 5 2.54,-1.27; 6 2.54,1.27
SCREWTERMINAL-5MM-2 = drill 1.3 pad 2.032 square: 1 0,0 | drill 1.3 pad 2.032: 2 5,0
1X03 = drill 1.016 long: 1 -2.54,0; 2 0,0; 3 2.54,0
CDRH2D09 = smd 1.3 x 1.3: P$1 -1.5,0; P$2 1.5,0
LED5MM = drill 0.813 octagon: A -1.27,0; K 1.27,0
150141M173100 = smd 1.5 x 0.9: 1 1.55,0.85; 2 1.55,-0.85; 3 -1.55,0.85; 4 -1.55,-0.85
SOT23 = smd 1 x 1.4: 1 -0.95,-1.1; 2 0.95,-1.1; 3 0,1.1
DIP08 = drill 0.813 pad 1.6 octagon: 1 -3.81,-3.81; 2 -1.27,-3.81; 3 1.27,-3.81; 4 3.81,-3.81; 5 3.81,3.81; 6 1.27,3.81; 7 -1.27,3.81; 8 -3.81,3.81
SOP65P400X130-8N = smd 1.321 x 0.356: 1 -1.829,0.965; 2 -1.829,0.33; 3 -1.829,-0.33; 4 -1.829,-0.965; 5 1.829,-0.965; 6 1.829,-0.33; 7 1.829,0.33; 8 1.829,0.965
DHT11 = drill 0.5 pad 0.698 long: GND 0,-7.62; NC 0,-5.08; SIG 0,-2.54; VCC 0,0
TP20R = smd 2 x 2: TP 0,0
SOT23-5 = smd 0.55 x 1.2: 1 -0.95,-1.3; 2 0,-1.3; 3 0.95,-1.3; 4 0.95,1.3; 5 -0.95,1.3
SOT95P237X112-3N = smd 1.321 x 0.559: 1 -1.092,0.94; 2 -1.092,-0.94 | smd 1.321 x 0.508: 3 1.092,0
BLUETOOTH_SMD = smd 2 x 1: 1 0,0; 2 0,-1.5; 3 0,-3; 4 0,-4.5; 5 0,-6; 6 0,-7.5; 7 0,-9; 8 0,-10.5; 9 0,-12; 10 0,-13.5; 11 0,-15; 12 0,-16.5; 13 0,-18; 22 13,-18; 23 13,-16.5; 24 13,-15; 25 13,-13.5; 26 13,-12; 27 13,-10.5; 28 13,-9; 29 13,-7.5; 30 13,-6; 31 13,-4.5; 32 13,-3; 33 13,-1.5; 34 13,0 | smd 1 x 1.8: 14 1.25,-19.75; 15 2.75,-19.75; 16 4.25,-19.75; 17 5.75,-19.75; 18 7.25,-19.75; 19 8.75,-19.75; 20 10.25,-19.75; 21 11.75,-19.75
QFN-10_PAD = smd 0.297 x 0.85: 1 -1,-1.475; 2 -0.5,-1.475; 3 0,-1.475; 4 0.5,-1.475; 5 1,-1.475; 6 1,1.475; 7 0.5,1.475; 8 0,1.475; 9 -0.5,1.475; 10 -1,1.475 | smd 0.7 x 0.28: 11 -1.5,0.25; 12 -1.5,-0.25; 13 1.5,0.25; 14 1.5,-0.25 | smd 2.4 x 1.65: 15 0,0
MICRO-USB-B = smd 0.4 x 1.4: D+ 0,2.85; D- 0.65,2.85; GND -1.3,2.85; ID -0.65,2.85; VBUS 1.3,2.85 | smd 2.3 x 1.9: GND@1 -3.75,0; GND@4 3.75,0 | smd 1.8 x 1.9: GND@2 1.15,0; GND@3 -1.15,0

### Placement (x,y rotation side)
BLDR-EN  54.93,11.43 0 top
C1  28.89,8.57 270 bottom
C2  50.48,22.23 270 bottom
C3  not placed on the board
C4  58.74,34.29 90 bottom
C5  56.83,41.27 270 bottom
C8  15.56,23.5 270 bottom
C9  7.94,18.73 180 bottom
C10  6.35,36.83 90 bottom
C11  16.83,36.2 180 top
C12  12.06,26.99 0 bottom
C13  18.41,33.34 90 bottom
C14  12.38,17.78 180 bottom
C17  57.15,43.81 180 top
C18  59.37,41.27 90 bottom
C19  51.75,41.27 270 top
C20  53.98,43.81 180 top
C21  54.29,41.27 90 bottom
C22  not placed on the board
C23  not placed on the board
C24  60.96,17.14 90 bottom
C25  65.72,40.01 0 bottom
C26  not placed on the board
C27  not placed on the board
C28  not placed on the board
C29  44.45,24.77 180 bottom
C30  44.45,22.86 180 bottom
C31  not placed on the board
C32  not placed on the board
C33  not placed on the board
C34  not placed on the board
C35  not placed on the board
C36  not placed on the board
C37  not placed on the board
C38  not placed on the board
C39  43.81,37.78 270 top
C40  41.91,44.77 0 bottom
C41  not placed on the board
C42  not placed on the board
DN1  8.26,29.7 90 top
DN2  7.94,18.73 90 top
IC1  39.05,48.26 180 top
IC2  55.56,28.57 90 top
IC3  55.56,49.53 0 top
JP1  11.11,43.18 45 top
JP2  18.41,12.38 0 top
JP3  55.24,3.49 0 top
JP9  16.83,48.26 135 top
L2  20.32,25.72 90 top
LED1  28.26,55.88 180 top
LED2  25,30 180 top
Q3  50.48,22.23 270 top
Q4  28.89,8.57 270 top
Q5  12.38,17.14 0 top
Q6  60.96,17.14 90 top
Q7  65.72,40.01 180 top
R2  7.62,34.29 180 top
R3  55.56,33.66 0 top
R4  50.48,52.7 90 top
R5  8.89,36.83 270 bottom
R6  50.48,49.53 90 top
R7  50.48,46.35 90 top
R8  16.83,34.29 0 top
R9  60.64,46.35 270 top
R10  32.7,54.93 270 top
R11  13.65,34.29 0 top
R12  12.7,26.35 270 top
R13  60.64,49.53 270 top
R14  60.64,52.7 270 top
R15  49.21,19.68 180 top
R16  50.16,11.75 0 top
R17  12.7,29.53 270 top
R18  48.58,49.53 90 top
R19  12.38,15.88 0 bottom
R20  20,34.92 180 top
R21  21.59,31.75 90 top
R22  47.94,45.09 0 top
R23  49.21,43.5 180 bottom
R24  55.56,55.24 0 top
R25  54.29,41.27 270 top
R26  24.45,33.66 270 top
R27  28.57,29.84 270 top
R28  27.94,33.02 180 top
R29  49.85,41.27 270 top
R30  59.37,41.27 270 top
R31  56.83,41.27 270 top
R32  61.28,28.89 270 top
R33  54.29,23.5 180 top
R34  57.47,23.5 180 top
R35  48.58,54.93 90 top
R38  68.9,25.08 270 bottom
R39  64.45,13.97 0 top
R40  61.28,13.97 0 top
R41  71.44,38.1 0 top
RESET  54.93,18.1 180 top
S3  25,20 270 top
S4  25,40 90 top
ST  9.21,23.5 180 top
SV2  72.71,35.56 90 bottom
TP1  58.74,33.66 90 top
TP2  50.48,26.67 90 top
TP3  11.11,20.32 0 top
TP4  18.1,38.73 0 top
TP5  51.44,34.61 270 top
TP6  68.26,14.61 0 top
U1  7.62,36.83 270 top
U2  46.04,54.93 180 top
U3  45.4,9.84 180 top
U6  16.51,28.26 0 top
X1  1,30 270 top

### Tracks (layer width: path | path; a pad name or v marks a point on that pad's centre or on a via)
3.3V1
  Top 0.305: U6.10 14.49,29.73 13.34,28.57 12.75,28.57 R17.2
  Top 0.508: R17.2 R12.1
435
  Top 0.406: LED2.3 28.37,29.15 R27.2
+3V3  (via drill 0.6)  (16 unrouted)
  Top 0.305: v15.56,25.72 16.01,26.17 U6.2 | R12.2 15.29,25.45 v15.56,25.72 | v15.56,25.72 15.24,25.4
  Top 0.406: IC3.4 47.62,49.53 46.49,50.66 IC1.9 | 72.39,35.88 72.39,38.05 R41.2 | U3.12 43.8,26.34 v43.5,26.04
  Top 0.508: 38.56,50.66 37.45,51.77 IC1.19 37.47,54.07 37.47,55.56 38.73,56.83 47.94,56.83 48.58,56.2 R35.2 49.58,56.83 66.99,56.83 72.39,51.44 72.39,35.88 SV2.VCC | IC1.9 38.56,50.66 | 37.78,46.99 37.78,49.88 38.56,50.66 | 37.78,46.99 36.65,45.86 IC1.31 30.62,45.86 28.89,44.13 28.89,36.51 26.04,33.66 26.04,32.7 25.08,31.75 25.08,30.16 24.07,29.15 LED2.1 23.45,25.99 21.91,24.45 21.91,21.91 21.27,21.27 15.24,21.27 | 37.78,46.99 39.05,45.72 IC1.39 39.05,39.37 47.94,30.48 | ST.8 8.27,22.53 10.48,20.32 TP3.TP 14.29,20.32 | 12.65,25.4 R12.2 | 14.29,20.32 15.88,18.73 JP2.2 | 14.29,20.32 15.24,21.27 | 15.24,25.4 15.24,21.27 | 47.94,30.48 53.1,30.48 IC2.8 | 47.94,30.48 47.31,29.84 47.31,26.99 46.67,26.35 | 46.67,26.35 45.41,26.35 U3.12 46.66,26.34 46.67,26.35 | R15.2 48.31,19.95 47.31,20.95 47.31,25.72 46.67,26.35
  Bottom 0.305: v15.56,25.72 C8.1
  Bottom 0.406: v43.5,26.04 43.5,24.82 C29.1 C30.1
ADC1  (via drill 0.6)
  Top 0.406: v44.45,42.23 43.28,42.23 IC1.44
  Bottom 0.406: R23.1 48.26,43.5 46.99,42.23 v44.45,42.23
ADC2  (via drill 0.6)
  Top 0.406: IC1.1 45.91,44.26 v46.35,43.81 | v55.24,53.02 55.24,54.66 R24.1
  Bottom 0.406: v46.35,43.81 46.99,43.81 55.24,52.07 v55.24,53.02
ADC3
  Top 0.406: R22.1 44.88,45.09 IC1.2
ADC4
  Top 0.406: R18.1 48.58,46.67 47.94,46.04 46.04,46.04 45.86,45.86 IC1.3
B  (via drill 0.6)
  Top 0.406: R26.1 25.35,34.55 v26.04,35.24 | IC1.20 36.65,56.38 v36.2,56.83
  Bottom 0.406: v26.04,35.24 32.7,41.91 32.7,55.24 34.29,56.83 v36.2,56.83
B2
  Top 0.406: R26.2 24.18,32.76 24.18,31.58 LED2.2 23.5,30.89
BLDR-EN  (via drill 0.6)
  Top 0.406: v36.83,48.26 IC1.28 | R16.1 49.27,10.21 v47.62,8.57
  Bottom 0.406: v36.83,48.26 38.1,48.26 38.42,47.94 38.42,13.65 43.5,8.57 v47.62,8.57
BT-EN  (1 unrouted)
C-STAT
  Top 0.406: R2.2 6.03,34.29 5.08,35.24 5.08,37.47 5.4,37.78 U1.1
D+  (via drill 0.6)
  Top 0.406: DN1.6 7.3,30.4 7.03,30.12 | X1.D+ 6.91,30 7.03,30.12 | v11.11,30.8 10.16,29.84 7.3,29.84 7.03,30.12 | v28.89,48.9 31.75,48.9 31.91,49.06 IC1.27
  Bottom 0.406: v11.11,30.8 v28.89,48.9
D-  (via drill 0.6)
  Top 0.406: X1.D- 6.84,29.35 7.3,28.89 DN1.1 7.3,28.89 7.62,29.21 10.79,29.21 v11.11,29.53 | v31.43,49.85 33.24,49.85 IC1.26
  Bottom 0.406: v11.11,29.53 v31.43,49.85
DATA-DHT  (via drill 0.6)
  Top 0.406: SV2.SIG 70.54,35.93 R41.1 70.54,46.3 v60.96,55.88 | v43.18,55.56 43.18,54.19 IC1.12
  Bottom 0.406: v60.96,55.88 43.5,55.88 v43.18,55.56
DEBUG-RX  (via drill 0.6)
  Top 0.406: JP9.2 18.1,49.53 26.35,49.53 v29.53,46.35 | IC1.32 33.23,45.09 31.43,45.09 v31.11,44.77
  Bottom 0.406: v31.11,44.77 v29.53,46.35
DEBUG-TX  (via drill 0.6)
  Top 0.406: JP9.1 18.62,46.56 20.32,48.26 26.04,48.26 v28.89,45.4 | v30.48,43.81 32.81,43.81 IC1.33
  Bottom 0.406: v28.89,45.4 v30.48,43.81
G  (via drill 0.6)
  Top 0.406: R28.1 28.84,33.28 v29.53,33.97 | v35.56,55.88 35.88,55.56 35.88,54.09 IC1.21
  Bottom 0.406: v29.53,33.97 29.53,37.47 33.66,41.59 33.66,54.93 34.61,55.88 v35.56,55.88
G2
  Top 0.406: R28.2 27.04,31.34 LED2.4
GND  (63 unrouted)
GND1
  Top 0.305: U6.9 16.01,30.34 15.56,30.8 13.07,30.8 R17.1 12.7,30.48 13.02,30.8 13.02,33.39 R11.1
HY-EN  (1 unrouted)
LED
  Top 0.406: R10.2 32.7,52.81 IC1.23
LIGHT/WAKEUP-BUTTON1  (via drill 0.6)
  Top 0.406: S4.T4 S4.T3 25.15,36.9 v25.08,36.83 | DN2.3 8.74,20.47 v8.26,20.95 | 11.02,23.81 10.48,23.81 v9.21,23.81 9.22,23.82 ST.3 11.02,23.81 | v13.34,23.81 11.02,23.81
  Bottom 0.406: v8.26,20.95 8.26,22.86 v9.21,23.81 | v25.08,36.83 14.61,26.35 14.61,25.08 v13.34,23.81
N$1
  Top 0.406: IC3.2 50.75,52.07 R4.1 R6.2
N$2
  Top 0.406: R6.1 R7.2 50.75,46.99 IC3.6
N$4
  Top 0.508: Q4.3 33.97,8.57 34.61,9.21 34.61,26.99 34.45,27.15 | 34.45,27.15 33.97,27.62 32.62,27.62 U3.22 32.4,28.34 U3.21 | U3.13 35.15,27.84 34.45,27.15
N$5
  Top 0.406: BLDR-EN.T4 BLDR-EN.T3 51.75,9.65 51.75,11.43 51.44,11.75 R16.2
N$6
  Top 0.406: R10.1 29.58,55.83 LED1.A
N$7
  Top 0.406: IC3.9 60.38,46.99 R9.1 R13.2
N$8
  Top 0.305: U6.3 16.51,24.13 16.83,23.81 20.55,23.81 L2.P$1
N$9  (via drill 0.6)
  Top 0.305: v13.97,26.99 15.3,26.99 U6.1
  Bottom 0.305: C12.1 v13.97,26.99
N$10  (2 unrouted)
  Top 0.406: DN2.2 6.35,18.73 6.03,18.41 6.03,17.78 7.62,16.19 11.16,16.19 R19.2 11.48,15.99 Q5.1
N$11  (1 unrouted)
N$12
  Top 0.406: R13.1 R14.2 60.38,52.07 IC3.13
N$14
  Top 0.406: IC3.1 50.75,53.34 R4.2 48.58,51.7 R18.2
N$15
  Top 0.406: IC3.7 50.75,45.72 R7.1 50.11,45.09 R22.2
N$19  (via drill 0.6)
  Top 0.406: IC3.8 60.38,45.72 R9.2 v60.64,44.13
  Bottom 0.406: R23.2 60.01,43.5 v60.64,44.13
N$21
  Top 0.406: R14.1 58.29,53.6 IC3.14 56.46,54.9 R24.2
N$22  (1 unrouted)
  Top 0.406: IC3.10 57.15,48.26 56.52,47.62 56.52,45.35 C17.1 58.05,43.5 C18.2
N$23
  Top 0.406: R33.1 R34.2 56.57,25.74 IC2.3
N$25
  Top 0.406: IC3.5 53.98,48.26 54.61,47.62 54.61,45.35 C20.2 53.08,43.5 C19.1 R29.1
N$26  (1 unrouted)
  Top 0.406: IC3.3 54.93,50.8 55.24,50.48 55.24,44.19 C20.1 54.88,42.76 R25.1
N$27  (1 unrouted)
  Top 0.406: IC3.12 56.2,50.8 55.88,50.48 55.88,44.19 C17.2 56.25,42.76 R31.1
N$28
  Top 0.508: R38.2 73.98,26.35 74.3,26.04 74.3,16.19 72.71,14.61 TP6.TP 67.94,14.61 | 67.94,14.61 67.31,13.97 R39.2 | 67.94,14.61 68.26,14.92 68.26,11.51 JP3.2
N$29
  Top 0.508: R38.7 60.33,26.35 60.01,26.04 60.01,17.29 Q6.3 59.86,14.49 R40.1
N$30
  Top 0.406: Q7.3 65.72,36.2 SV2.GND
N$33
  Top 0.406: 62.23,33.34 61.28,34.29 61.28,40.01 60.91,40.38 R30.2 58.47,41.27 50.48,41.27 49.85,40.64 R29.2 | 62.23,33.34 72.39,33.34 72.71,33.02 R38.1 | 62.23,33.34 61.28,32.38 R32.1
N$34
  Top 0.406: R25.2 54.03,40.38 54.03,36.56 52.07,34.61 | TP5.TP 52.07,34.61 | 52.07,34.61 53.98,32.7 54.61,32.7 54.93,32.38 IC2.7 54.93,29.84 56.78,27.99 R32.2
N$35
  Top 0.406: R38.8 57.47,28.89 56.2,30.16 IC2.6 56.2,33.39 R3.2 56.46,40.01 R31.2
PAD@4  (via drill 0.6)
  Top 0.305: U6.12 U6.11 15.81,28.51 15.88,28.57 16.19,28.26 U6.15 | U6.13 U6.14 | U6.13 16.76,28.51 U6.15 | U6.15 17.01,27.76 U6.4 17.01,26.17 17.78,25.4 v17.78,24.77 | U6.13 18.66,28.51 v19.05,28.89 | v20.32,30.16 20.95,30.8 21.54,30.8 R21.1
  Top 0.508: Q5.3 12.38,18.41 13.02,19.05 v13.65,19.05
  Bottom 0.305: v19.05,28.89 v20.32,30.16
  Bottom 0.508: v13.65,19.05 14.61,19.05 17.78,22.23 v17.78,24.77
PDI_DATA  (via drill 0.6)
  Top 0.406: IC1.34 35.05,36.64 v34.92,36.51 | v25.08,15.24 17.78,15.24 17.14,14.61 17.14,12.06 16.19,11.11 JP2.1
  Bottom 0.406: v25.08,15.24 26.04,15.24 34.92,24.13 v34.92,36.51
R  (via drill 0.6)
  Top 0.406: R27.1 29.16,30.75 v30.48,32.07 | v34.92,51.75 34.92,53.93 IC1.22
  Bottom 0.406: v30.48,32.07 30.48,37.15 34.61,41.27 34.61,51.44 v34.92,51.75
RST/PDI_CLK  (via drill 0.6)
  Top 0.406: RESET.T3 RESET.T4 50.38,19.95 R15.1 50.16,19.63 50.16,8.57 47.31,5.71 26.04,5.71 20.95,10.79 JP2.5 v23.18,13.34 | IC1.35 35.85,40.98 v35.88,40.96
  Bottom 0.406: v35.88,40.96 35.88,22.54 26.67,13.34 v23.18,13.34
RX-TX(BT)  (via drill 0.6)
  Top 0.406: v42.86,11.11 44.13,9.84 U3.1 | IC1.16 39.85,52.23 v39.69,52.07
  Bottom 0.406: v42.86,11.11 39.69,14.29 v39.69,52.07
SEN1-EN  (1 unrouted)
SEN2-EN  (1 unrouted)
SEN-GND  (via drill 0.6)
  Top 0.508: Q3.3 52.07,22.23 | 52.07,22.23 58.1,22.23 58.42,22.54 58.42,23.44 R34.1 58.37,25.21 IC2.4 | U2.2 47.13,55.1 47.31,54.93 v51.44,54.93 | IC3.11 v61.91,49.53 | v51.75,24.13 51.75,22.54 52.07,22.23 | v54.61,34.92 54.61,33.71 R3.1
  Bottom 0.508: v51.44,54.93 58.42,54.93 62.23,51.12 62.23,49.85 v61.91,49.53 62.23,49.21 62.23,40.32 56.83,34.92 v54.61,34.92 53.34,34.92 51.44,36.83 49.85,36.83 47.94,34.92 47.94,32.7 52.39,28.26 52.39,24.77 v51.75,24.13
TX-RX(BT)  (via drill 0.6)
  Top 0.406: v40.32,55.88 39.69,55.88 39.05,55.24 IC1.17 | U3.2 44.22,11.34 v43.18,12.38
  Bottom 0.406: v40.32,55.88 41.91,54.29 41.91,13.65 v43.18,12.38
UVLO1  (via drill 0.6)
  Top 0.305: U6.7 17.01,31.57 v16.83,31.75 | v14.92,31.75 14.61,32.07 14.61,34.24 R11.2
  Top 0.508: R11.2 R8.1 C11.2
  Bottom 0.305: v16.83,31.75 v14.92,31.75
V-B  (via drill 0.6)  (1 unrouted)
  Top 0.305: U6.5 17.71,26.99 20.09,26.99 L2.P$2 20,27.54 20,29.21 19.48,29.73 U6.6 17.51,30.84 17.78,31.11 | U6.8 16.51,30.8 15.88,31.43 15.88,32.07 16.51,32.7 17.46,32.7 | 17.46,32.7 17.78,33.02 17.78,33.6 R8.2 | 17.78,31.11 17.78,32.38 17.46,32.7 | 17.78,31.11 18.1,31.11 v18.41,31.43
  Top 0.406: S4.T2 S4.T1 21.08,36.9 R20.2 | S3.T1 S3.T2
  Top 0.508: U1.3 7.3,35.88 7.62,36.2 7.62,38.42 9.84,40.64 12.24,40.64 JP1.1 13.17,39.86 15.24,37.78 17.14,37.78 | TP4.TP 17.14,37.78 | 17.14,37.78 17.14,37.47 17.78,36.83 17.78,36.25 C11.1 R8.2 18.47,34.29 R20.2 | L2.P$2 22,27.22 v22.23,26.99 | v26.99,25.72 26.99,23.24 S3.T1
  Bottom 0.305: v18.41,31.43 C13.1
  Bottom 0.508: v22.23,26.99 25.72,26.99 v26.99,25.72
V-BATT  (via drill 0.6)
  Top 0.406: R20.1 20.95,34.29 21.59,33.66 R21.2 21.64,32.7 v23.18,32.7 | IC1.41 40.64,40.32 v40.96,40.01 | v33.97,33.66 36.83,36.51 v40.64,36.51
  Bottom 0.406: v33.97,33.66 30.48,30.16 25.72,30.16 v23.18,32.7 | v40.96,40.01 40.96,36.83 v40.64,36.51
V-BATT-H  (via drill 0.6)
  Top 0.406: R40.2 R39.1 63.5,14.02 v63.5,16.51 | IC1.42 41.45,40.78 41.59,40.64 44.13,40.64 v49.53,35.24
  Bottom 0.406: v63.5,16.51 62.55,17.46 62.55,19.37 49.85,32.07 49.85,34.92 v49.53,35.24
V-REF  (via drill 0.6)  (2 unrouted)
  Top 0.406: IC2.1 IC2.2 v54.93,28.26 | C4.1 57.47,32.12 IC2.5 58.81,31.04 59.05,30.8 v59.05,30.16 | 44.45,38.73 40.96,38.73 39.85,39.84 IC1.40 | v50.8,32.38 44.45,38.73 | C39.1 44.4,38.68 44.45,38.73
  Bottom 0.406: v59.05,30.16 59.05,29.53 58.1,28.57 55.24,28.57 v54.93,28.26 v50.8,32.38
V-REF-B  (via drill 0.6)
  Top 0.406: R35.1 47.62,54.03 | 47.62,54.03 47.17,54.03 U2.1 | R33.2 53.39,23.76 TP2.TP v49.21,27.94 | v43.18,45.72 43.18,46.35 43.5,46.67 44.84,46.67 IC1.4 47.3,46.66 v47.62,46.99 | v47.62,52.7 47.62,54.03
  Bottom 0.406: v49.21,27.94 43.18,33.97 43.18,44.77 | 43.18,44.77 v43.18,45.72 | v47.62,46.99 v47.62,52.7 | C40.1 43.18,44.77
VUSB  (1 unrouted)
  Top 0.508: 7.3,32.38 3.17,32.38 2.54,31.75 2.54,28.89 2.73,28.7 X1.VBUS 4.96,28.7 5.08,28.57 5.08,24.45 5.71,23.81 | 7.3,32.38 8.26,31.43 DN1.5 | 7.3,32.38 8.57,33.66 8.57,34.24 R2.1 8.52,35.48 U1.4 | 5.71,23.81 5.4,23.5 5.4,21.12 DN2.4 | 5.71,23.81 7.37,23.81 ST.6
WAKEUP-BUTTON1  (via drill 0.6)
  Top 0.406: S3.T3 S3.T4 23.08,16.83 v21.27,16.83 | DN2.1 9.83,18.08 v9.84,18.1 | v12.38,22.54 11.05,22.54 ST.1
  Bottom 0.406: v21.27,16.83 16.19,16.83 13.65,14.29 10.79,14.29 10.16,14.92 10.16,17.78 v9.84,18.1 13.02,21.27 13.02,21.91 v12.38,22.54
